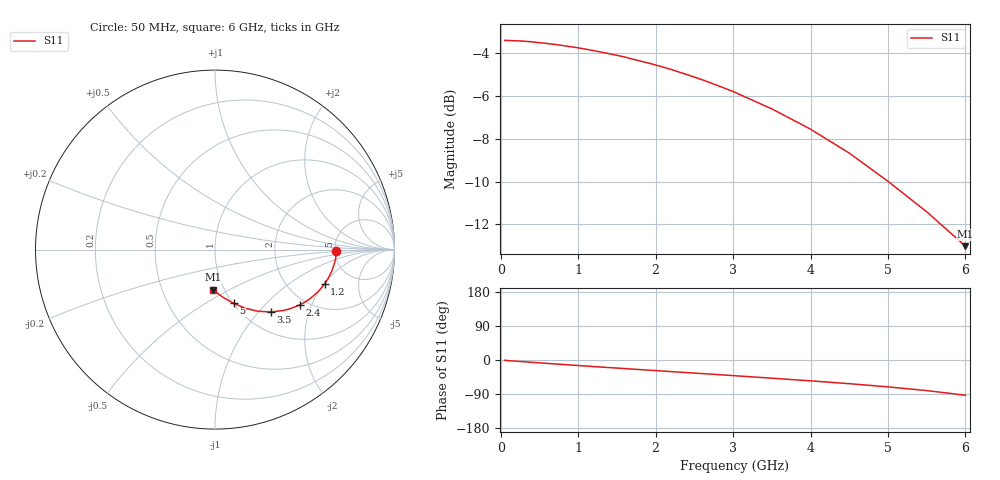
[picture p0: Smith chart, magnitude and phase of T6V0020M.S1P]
! SIEMENS Discrete & RF Semiconductors
! BAT62
! Si Schottky Diode in SOT143
! IF = 20 mA
! S-Parameters:  February  1997
# GHz  S  MA  R  50
!  f  S11
! GHz  MAG  ANG
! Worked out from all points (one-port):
!   34 points, 50 MHz to 6 GHz, reference 50 ohm
!   lowest |S11| = -13.0 dB at 6 GHz (marker M1), VSWR 1.58, Z = 44.3 - j20.8 ohm
!   |S11| at or under -10 dB: 5.006 GHz to end of sweep
!   S11 on the Smith chart (normalised r, x): 50 MHz: 5.16, -0.16; 1.2 GHz: 3.15, -2.03; 2.4 GHz: 1.82, -1.64; 3.5 GHz: 1.32, -1.17; 5 GHz: 1.01, -0.67; 6 GHz: 0.89, -0.42
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0.05  0.6758 -0.7
0.1  0.6758 -1.6
0.15  0.6751 -2.4
0.2  0.6745 -3.1
0.25  0.6741 -3.9
0.4  0.6708 -6.1
0.6  0.6647 -8.9
0.7  0.6616 -10.4
0.8  0.6576 -11.8
1  0.6495 -14.6
1.2  0.6397 -17.3
1.3  0.6345 -18.7
1.4  0.6295 -20.0
1.6  0.6183 -22.7
1.7  0.6112 -24.0
1.9  0.599 -26.6
2  0.5923 -28.0
2.2  0.5783 -30.6
2.4  0.5627 -33.2
2.6  0.5472 -35.8
2.8  0.5305 -38.5
3  0.5135 -41.2
3.5  0.4678 -48.0
4  0.4194 -55.0
4.5  0.3688 -62.5
5  0.3168 -70.9
5.5  0.269 -80.7
6  0.2235 -93.0
